PROGRAM RotaryKnifeCamTable
VAR_INPUT
	Execute : BOOL;
	ProductLength : LREAL;
END_VAR
VAR_OUTPUT
	Done : BOOL;
	Busy : BOOL;
END_VAR
VAR
	state: INT;
	TriggerExecute: R_TRIG;
	ReadMotionFunction: MC_ReadMotionFunction;
	CamData : ARRAY[1..MAXCAMPOINTS] OF MC_MotionFunctionPoint;
	CamRef : MC_CAM_REF;
	RotaryKnifeSynchronousRange: LREAL;
	WriteMotionFunction: MC_WriteMotionFunction;
	lrSlavepos: LREAL;
	
	fbPosTrig:Tc2_Standard.R_TRIG;
END_VAR
VAR CONSTANT
	MAXCAMPOINTS 			: UDINT := 10;
END_VAR

(*
	modification of a rotary knife electronic cam table 
	for use with varying product length
 *)
TriggerExecute(CLK:=Execute);



fbPosTrig(CLK:= VirtualWeb.NcToPlc.ModuloActPos>0 AND VirtualWeb.NcToPlc.ModuloActPos<2);

IF fbPosTrig.Q THEN
	IF lrSlavePos<=180 AND lrSlavePos>=100 THEN
	lrSlavePos:=lrSlavePos-10;
	ELSE
	lrSlavePos:=180;	
	END_IF
END_IF


CASE state OF
	0 : 	(* init *)
		Busy := FALSE;
		IF NOT Execute THEN
			Done := FALSE;
		END_IF
		IF TriggerExecute.Q THEN
			Busy := TRUE;
			CamRef.ArraySize := SIZEOF(CamData);
			CamRef.pArray := ADR(CamData);
			CamRef.NoOfColumns := 1; (* allways 1 for motion functions *)
			CamRef.NoOfRows := MAXCAMPOINTS;
			ReadMotionFunction.Execute := FALSE;
			WriteMotionFunction.Execute := FALSE;
			state := state + 1;
		END_IF

	1 : 	(* read cam data *)
		ReadMotionFunction.Execute := TRUE;
		
		
		
		
		IF ReadMotionFunction.Done THEN
			state := state + 1;
		END_IF

	2 : 	(* modify points of cam table *)
		(*
			point 1 is allways at 0;0 (cutting position)
			point 2 and 3 have to be modified corresponding to the product length (synchonous range)
		*)
		
		CamData[1].SlaveVelo := ProductLength / ROTARYKNIFECIRCUMFERENCE;
		
		RotaryKnifeSynchronousRange := CamData[2].SlavePos;
		CamData[2].MasterPos := RotaryKnifeSynchronousRange / ProductLength * ROTARYKNIFECIRCUMFERENCE;
		CamData[2].SlaveVelo := ProductLength / ROTARYKNIFECIRCUMFERENCE;

		RotaryKnifeSynchronousRange := 360 - CamData[3].SlavePos;
		CamData[3].MasterPos := 360 - RotaryKnifeSynchronousRange / ProductLength * ROTARYKNIFECIRCUMFERENCE;
		CamData[3].SlaveVelo := ProductLength / ROTARYKNIFECIRCUMFERENCE;

		
		WriteMotionFunction.Execute := TRUE;
		IF WriteMotionFunction.Done THEN
			Done := TRUE;
			Busy := FALSE;
			state := 0;
		END_IF

END_CASE

ActCamTable();

ACTION ActCamTable:
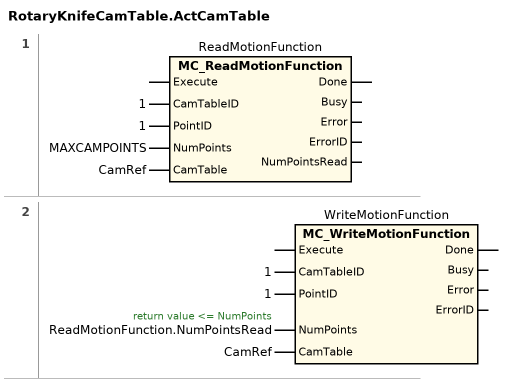
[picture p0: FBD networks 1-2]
// NETWORK 1
ReadMotionFunction(CamTableID := 1, PointID := 1, NumPoints := MAXCAMPOINTS, CamTable := CamRef); // MC_ReadMotionFunction

// NETWORK 2
//   ReadMotionFunction.NumPointsRead: return value <= NumPoints
WriteMotionFunction(
    CamTableID := 1,
    PointID := 1,
    NumPoints := ReadMotionFunction.NumPointsRead,
    CamTable := CamRef); // MC_WriteMotionFunction
END_ACTION

END_PROGRAM
